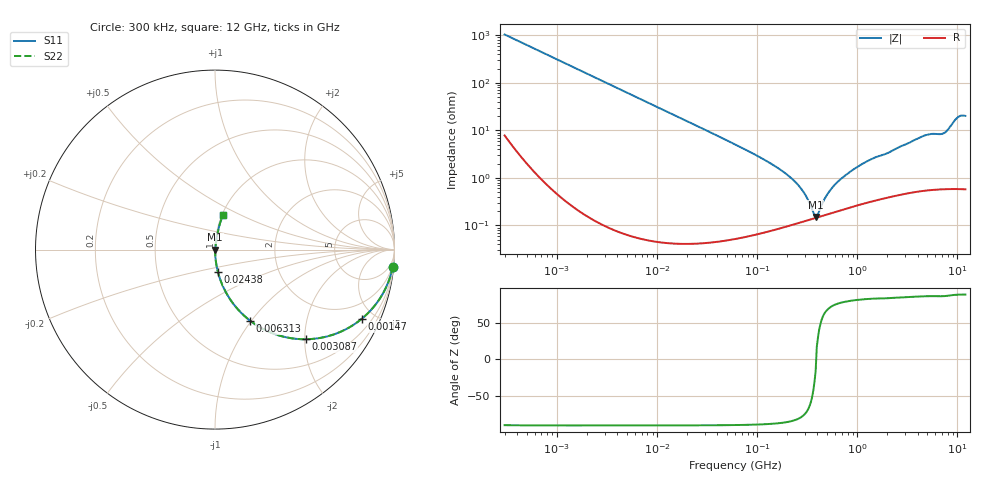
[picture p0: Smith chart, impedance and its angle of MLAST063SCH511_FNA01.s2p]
! MLAST063SCH511_FNA01  S-PARAMETER MODEL  ( General Type )
! Model Generated by TAIYO YUDEN Corporation (http://www.ty-top.com)
! Version 1.0
! TAIYO YUDEN Control No. 160830
! Copyright(c) 2016 TAIYO YUDEN CO.,LTD. All Rights Reserved.
! Product Description (link to TY-COMPAS)
! https://ds.yuden.co.jp/TYCOMPAS/or/detail?pn=MLAST063SCH511JFNA01&u=M
! Products Name : Multilayer Ceramic Capacitors
! Characteristics :
!  Capacitance : 510 pF , Rated Voltage : 25V , TCC : CH / C0H
!  Case Size : 0.6 x 0.3 / 0.024 x 0.012 [mm/inch] , Thickness : 0.3 / 0.012 [mm/inch]
!  (Conditions: Temperature = 25 degC , DC Bias Current/Voltage = 0A / 0V)
! External Node Assignments :
!  1  o---| |---o  2
! GND o---------o GND
! Frequency Range : 0.3MHz  -  12000MHz  [ 401 STEP ]
# MHz S RI R 50
! Freq[MHz].  S11 Real  S11 Imag  S21 Real  S21 Imag  S12 Real  S12 Imag  S22 Real  S22 Imag
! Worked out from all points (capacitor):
!   401 points, 300 kHz to 12 GHz, reference 50 ohm
!   read as one part in series: C = 510 pF near 316.3 kHz
!   lowest |Z| = 150 mohm at 383.3 MHz (marker M1)
!   series resonance near 388.2 MHz, so ESL is about 330 pH
!   S11 on the Smith chart (normalised r, x): 300 kHz: 1, -21; 1.47 MHz: 1.00, -4.24; 3.087 MHz: 1.00, -2.02; 6.313 MHz: 1.00, -0.99; 24.38 MHz: 1.00, -0.26; 12 GHz: 1.01, +0.40
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0.3  0.9901 -0.0951  0.00986 0.0951  0.00986 0.0951  0.9901 -0.0951
0.778586  0.941 -0.2347  0.059 0.2347  0.059 0.2347  0.941 -0.2347
1.470382  0.818 -0.3852  0.182 0.3852  0.182 0.3852  0.818 -0.3852
1.769972  0.7564 -0.4288  0.2436 0.4288  0.2436 0.4288  0.7564 -0.4288
3.087269  0.5053 -0.4995  0.4947 0.4995  0.4947 0.4995  0.5053 -0.4995
6.312676  0.1966 -0.3969  0.8034 0.3969  0.8034 0.3969  0.1966 -0.3969
10.44266  0.0822 -0.274  0.9178 0.274  0.9178 0.274  0.0822 -0.274
24.37677  0.0164 -0.1254  0.9836 0.1254  0.9836 0.1254  0.0164 -0.1254
60  0.00309 -0.0506  0.9969 0.0506  0.9969 0.0506  0.00309 -0.0506
208.3979  0.0011 -0.0108  0.9989 0.0108  0.9989 0.0108  0.0011 -0.0108
286.3882  0.00122 -0.00511  0.9988 0.00511  0.9988 0.00511  0.00122 -0.00511
353.9943  0.00137 -0.00168  0.9986 0.00168  0.9986 0.00168  0.00137 -0.00168
383.2761  0.00144 -0.000419  0.9986 0.000419  0.9986 0.000419  0.00144 -0.000419
404.1309  0.00149 0.000845  0.9985 -0.000845  0.9985 -0.000845  0.00149 0.000845
512.9422  0.00176 0.00452  0.9982 -0.00452  0.9982 -0.00452  0.00176 0.00452
686.4755  0.00218 0.00929  0.9978 -0.00929  0.9978 -0.00929  0.00218 0.00929
1166.079  0.0033 0.0204  0.9967 -0.0204  0.9967 -0.0204  0.0033 0.0204
2088.533  0.00508 0.0341  0.9949 -0.0341  0.9949 -0.0341  0.00508 0.0341
4747.894  0.0114 0.0773  0.9886 -0.0773  0.9886 -0.0773  0.0114 0.0773
7254.098  0.013 0.0848  0.987 -0.0848  0.987 -0.0848  0.013 0.0848
9968.853  0.0382 0.1766  0.9618 -0.1766  0.9618 -0.1766  0.0382 0.1766
12000  0.0442 0.1918  0.9558 -0.1918  0.9558 -0.1918  0.0442 0.1918
